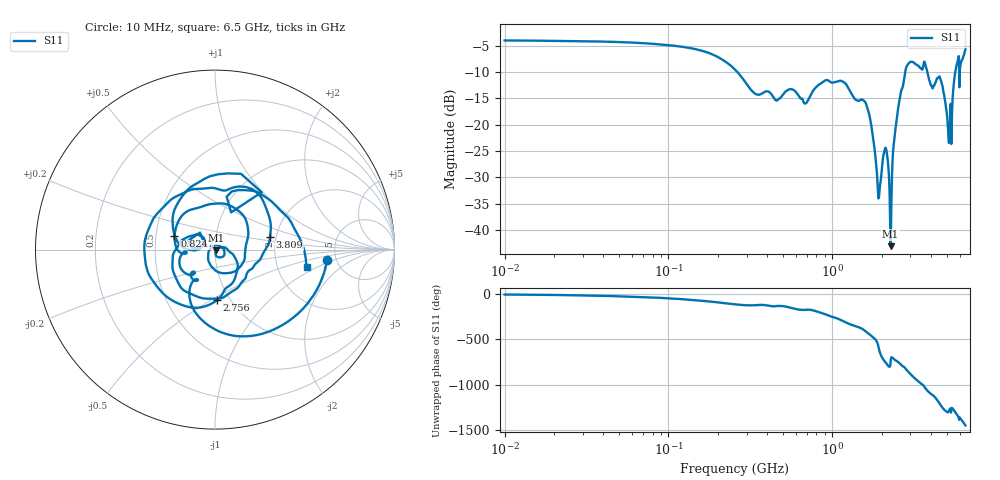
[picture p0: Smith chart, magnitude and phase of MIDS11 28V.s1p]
!Keysight Technologies,E5080B,MY59100498,A.17.05.10
!Date: Wednesday, August 30, 2023 14:18:05
!Correction: S11(C  1-Port  )
!S1P File: Measurement: S11:Log Frequency Sweep
# Hz S  dB  R 50
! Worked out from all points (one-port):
!   1601 points, 10 MHz to 6.5 GHz, reference 50 ohm
!   lowest |S11| = -43.0 dB at 2.269 GHz (marker M1), VSWR 1.01, Z = 50.5 - j0.505 ohm
!   |S11| at or under -10 dB: 263.1 MHz to 2.788 GHz (2.525 GHz wide, 166 % of centre); 3.805 GHz to 5.642 GHz (1.837 GHz wide, 38.9 % of centre); 5.957 GHz to 6.005 GHz (48.1 MHz wide, 0.804 % of centre)
!   S11 on the Smith chart (normalised r, x): 10 MHz: 4.21, -0.79; 824.7 MHz: 0.63, +0.10; 2.756 GHz: 0.87, -0.53; 3.809 GHz: 1.86, +0.28; 6.5 GHz: 2.92, -0.78
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1e7  -4.04 -5.2
2.256172e7  -4.13 -11.2
5.069748e7  -4.35 -24.4
1.139202e8  -5.13 -53.0
2.54951e8  -9.55 -113.4
3.453918e8  -14.27 -122.0
5.728895e8  -13.34 -155.7
6.873597e8  -15.98 -173.3
8.247023e8  -12.48 161.7
1.086041e9  -11.80 87.0
1.292537e9  -13.79 24.8
1.641229e9  -16.90 -67.2
1.92971e9  -33.73 110.6
2.1266e9  -24.50 -39.7
2.268898e9  -43.04 -45.2
2.440395e9  -20.45 -12.4
2.755512e9  -11.00 -87.7
2.904406e9  -8.50 -135.7
3.098749e9  -8.10 171.7
3.373695e9  -8.89 112.0
3.584899e9  -9.12 76.2
3.809325e9  -10.05 12.7
4.371419e9  -11.26 -88.7
4.645083e9  -12.01 -160.9
5.202588e9  -22.03 166.0
5.618531e9  -10.33 140.1
5.946149e9  -7.70 50.8
6.5e9  -5.69 -10.8
